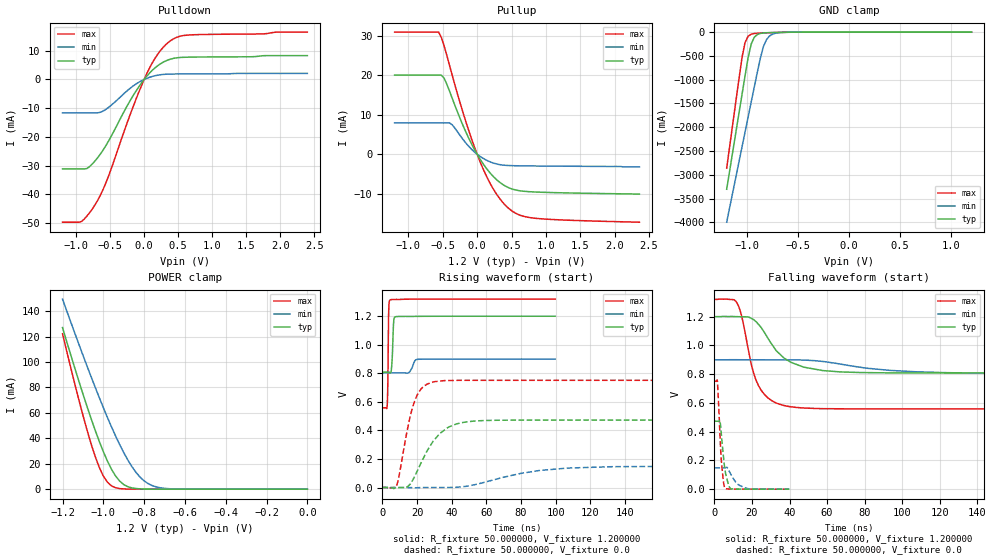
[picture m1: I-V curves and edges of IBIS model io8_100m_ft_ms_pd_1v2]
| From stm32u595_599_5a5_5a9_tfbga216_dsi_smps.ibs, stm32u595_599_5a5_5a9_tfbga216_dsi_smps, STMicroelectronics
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|   Model io8_100m_ft_ms_pd_1v2
[Model]  io8_100m_ft_ms_pd_1v2
Model_type I/O
Polarity   Non-Inverting
Enable   Active-Low
Vinl =   0.360000V
Vinh =   0.840000V
Vmeas =  0.600000V
Cref =   50.000000pF
Rref =   100.000000M
Vref =   0.0V
C_comp   2.947800pF   2.877700pF   2.996100pF
[Temperature Range]   25.000000   0.140000k   -40.000000
[Pullup Reference]   1.200000V   0.900000V   1.320000V
[Pulldown Reference]   0.0V   0.0V   0.0V
[POWER Clamp Reference]   1.200000V   0.900000V   1.320000V
[GND Clamp Reference]   0.0V   0.0V   0.0V
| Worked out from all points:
|   slope of the pulldown table from 0 to 0.18 V, typ, clamps not added: 40.7 ohm
|   slope of the pullup table from 0 to 0.18 V, typ, clamps not added: 39.5 ohm
|   GND clamp passes 1 mA (typ) near -0.51 V on its own axis
|   POWER clamp passes 1 mA (typ) near -0.86 V on its own axis
|   rising waveform, R_fixture 50.000000, V_fixture 1.200000: 20-80 % time 750ps typ, 2.06ns min, 441ps max; typ from 0.808 V to 1.2 V
|   rising waveform, R_fixture 50.000000, V_fixture 0.0: 20-80 % time 13.8ns typ, 33.6ns min, 7.83ns max; typ from 0 V to 0.472 V
|   falling waveform, R_fixture 50.000000, V_fixture 1.200000: 20-80 % time 15.2ns typ, 36.9ns min, 8.75ns max; typ from 1.2 V to 0.808 V
|   falling waveform, R_fixture 50.000000, V_fixture 0.0: 20-80 % time 2.49ns typ, 4.75ns min, 1.84ns max; typ from 0.472 V to 0 V
[Pulldown]
|Voltage   I(typ)   I(min)   I(max)
-1.2V     -31.16mA   -11.61mA   -49.71mA
-920mV    -31.16mA   -11.61mA   -49.48mA
-840mV    -31mA      -11.61mA   -47.54mA
-720mV    -28.33mA   -11.61mA   -43.58mA
-560mV    -22.95mA   -10.37mA   -35.89mA
-200mV    -7.146mA   -2.964mA   -11.89mA
0V        0A         0A         0A
160mV     4.047mA    1.298mA    7.361mA
360mV     6.87mA     1.87mA     13mA
480mV     7.543mA    1.91mA     14.69mA
640mV     7.765mA    1.923mA    15.46mA
2.4V      8.308mA    2.101mA    16.51mA
[Pullup]
|Voltage   I(typ)   I(min)   I(max)
-1.2V     20.06mA    7.936mA    30.97mA
-560mV    20.06mA    7.936mA    30.97mA
-480mV    19.26mA    7.936mA    27.49mA
-360mV    14.08mA    7.421mA    19.88mA
-160mV    5.494mA    2.768mA    8.045mA
40mV      -1.16mA    -508.1uA   -1.774mA
240mV     -5.73mA    -2.256mA   -8.953mA
360mV     -7.518mA   -2.715mA   -11.96mA
480mV     -8.639mA   -2.877mA   -14.04mA
640mV     -9.31mA    -2.942mA   -15.55mA
880mV     -9.601mA   -2.986mA   -16.29mA
2.36V     -10.1mA    -3.2mA     -17.23mA
[GND_clamp]
|Voltage   I(typ)   I(min)   I(max)
-1.2V     -3.305A    -3.998A    -2.862A
-1.05V    -1.316A    -2.418A    -539.3mA
-1.02V    -921mA     -2.103A    -218.8mA
-990mV    -539.5mA   -1.788A    -87.45mA
-960mV    -252.2mA   -1.474A    -44.37mA
-930mV    -110.5mA   -1.16A     -30.33mA
-870mV    -28.04mA   -549.1mA   -21.1mA
-840mV    -18.44mA   -305.6mA   -18.29mA
-810mV    -13.92mA   -159.7mA   -15.75mA
-780mV    -11.24mA   -82.36mA   -13.39mA
-600mV    -2.986mA   -4.279mA   -3.072mA
1.2V      30.28uA    18.17uA    37.27uA
[POWER_clamp]
|Voltage   I(typ)   I(min)   I(max)
-1.2V     127mA      149.4mA    122.2mA
-1.12V    84.97mA    114mA      70.27mA
-1.06V    55.51mA    88.42mA    35.67mA
-1.02V    37.63mA    72.04mA    17.17mA
-1V       29.51mA    64.13mA    10.3mA
-960mV    15.69mA    48.99mA    2.571mA
-900mV    3.624mA    28.77mA    182.8uA
-840mV    490.7uA    13.24mA    11.35uA
-800mV    116.8uA    6.532mA    1.77uA
-740mV    13.2uA     1.723mA    109.1nA
-620mV    167.3nA    79.35uA    0A
0V        0A         17.84nA    0A
[Ramp]
| variable   typ   min   max
dV/dt_r  0.28339/13.81887n   88.80588m/33.56225n 0.45045/7.81454n
dV/dt_f  0.23488/15.13762n   58.04400m/36.80260n 0.45673/8.73101n
R_load = 50.000000
[Rising Waveform]
R_fixture= 50.000000
V_fixture= 1.200000
V_fixture_min= 0.900000
V_fixture_max= 1.320000
|time   V(typ)   V(min)   V(max)
0s        808mV      802.7mV    558.2mV
2.803ns   808mV      802.7mV    574.3mV
3.203ns   808.1mV    802.7mV    762.8mV
3.604ns   807.9mV    802.7mV    1.21V
4.605ns   803.7mV    802.7mV    1.314V
5.405ns   851.1mV    802.7mV    1.316V
6.607ns   1.171V     802.7mV    1.316V
7.608ns   1.195V     802.7mV    1.317V
20.42ns   1.198V     897.3mV    1.319V
99.7ns    1.199V     899.4mV    1.319V
[Rising Waveform]
R_fixture= 50.000000
V_fixture= 0.0
V_fixture_min= 0.0
V_fixture_max= 0.0
|time   V(typ)   V(min)   V(max)
0s        2.143uV    1.131uV    2.528uV
8.408ns   -704.7uV   90.72nV    19.93mV
15.62ns   18.27mV    -741.6uV   474.7mV
18.62ns   77.46mV    -1.84mV    605mV
22.82ns   184.9mV    -261.9uV   696.6mV
30.03ns   334.1mV    -33.91uV   741.1mV
40.84ns   437.2mV    977.2uV    749.7mV
56.46ns   467.7mV    28.86mV    750.6mV
107.5ns   472.3mV    136.5mV    750.7mV
299.1ns   472.4mV    148.1mV    750.8mV
[Falling Waveform]
R_fixture= 50.000000
V_fixture= 1.200000
V_fixture_min= 0.900000
V_fixture_max= 1.320000
|time   V(typ)   V(min)   V(max)
0s        1.199V     899.4mV    1.319V
12.01ns   1.199V     900mV      1.295V
14.41ns   1.199V     899.7mV    1.208V
20.02ns   1.185V     899.6mV    847.5mV
23.22ns   1.149V     899.6mV    726.7mV
29.63ns   1.025V     899.2mV    623.2mV
40.84ns   881.8mV    899mV      572.6mV
67.27ns   815.1mV    869.4mV    558.7mV
123.3ns   807.9mV    810mV      558.2mV
398.8ns   808mV      802.7mV    558.2mV
[Falling Waveform]
R_fixture= 50.000000
V_fixture= 0.0
V_fixture_min= 0.0
V_fixture_max= 0.0
|time   V(typ)   V(min)   V(max)
0s        472.4mV    148.1mV    750.8mV
1.522ns   472.4mV    148.1mV    754.8mV
2.883ns   478.5mV    148.1mV    394.5mV
3.604ns   392.5mV    148.1mV    210.9mV
4.885ns   214.4mV    147.9mV    43.68mV
5.445ns   150.1mV    148.2mV    8.892mV
7.367ns   35.95mV    138.2mV    1.439mV
8.729ns   2.645mV    103.7mV    943.9uV
16.5ns    342.2uV    8.308mV    325.8uV
39.88ns   2.143uV    1.131uV    2.528uV
